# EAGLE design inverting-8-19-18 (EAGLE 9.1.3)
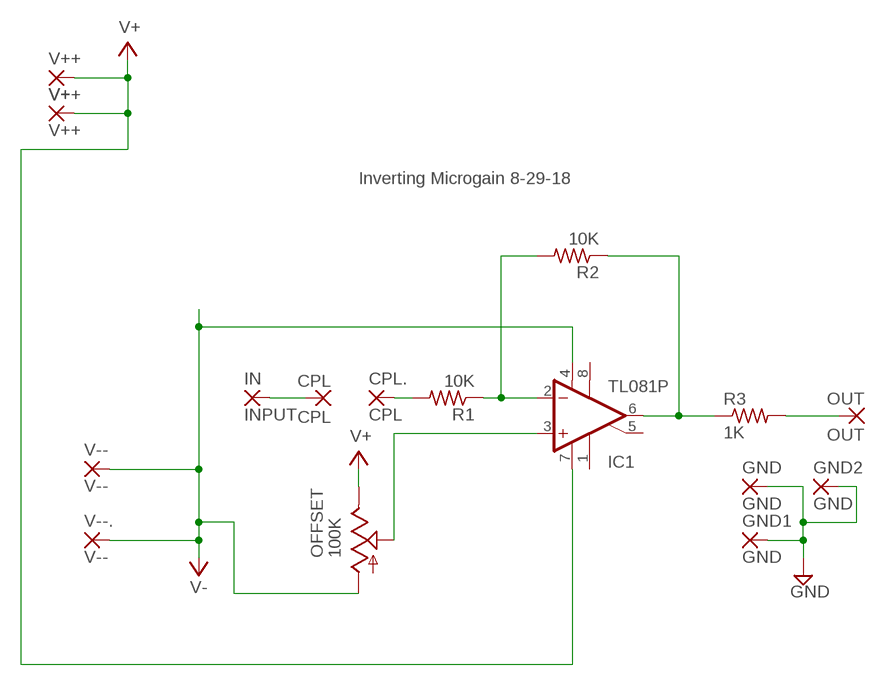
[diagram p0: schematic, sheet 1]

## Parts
CPL  CPL  3,17/1,3  [3,17/1,3]
CPL.  CPL  3,17/1,3  [3,17/1,3]
GND  GND  3,17/1,3  [3,17/1,3]
GND1  GND  3,17/1,3  [3,17/1,3]
GND2  GND  3,17/1,3  [3,17/1,3]
IC1  TL081P  [DIL08]
IN  INPUT  3,17/1,3  [3,17/1,3]
OFFSET  100K  TRIM_US-S63X  [S63X]
OUT  OUT  3,17/1,3  [3,17/1,3]
R1  10K  R-US_0204/7  [0204/7]
R2  10K  R-US_0204/7  [0204/7]
R3  1K  R-US_0204/7  [0204/7]
V+  V++  3,17/1,3  [3,17/1,3]
V++  V++  3,17/1,3  [3,17/1,3]
V--  V--  3,17/1,3  [3,17/1,3]
V--.  V--  3,17/1,3  [3,17/1,3]

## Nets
GND: GND1.1(P) GND2.1(P) GND.1(P)
N$1: IC1.3(+IN) OFFSET.S
N$3: CPL.1(P) IN.1(P)
N$4: CPL..1(P) R1.2
N$5: IC1.2(-IN) R1.1 R2.2
N$18: IC1.6(OUT) R2.1 R3.1
N$19: OUT.1(P) R3.2
V+: IC1.7(V+) OFFSET.E V++.1(P) V+.1(P)
V-: IC1.4(V-) OFFSET.A V--.1(P) V--..1(P)
Unconnected: IC1.1(ON1) IC1.5(ON2) IC1.8(OPT)

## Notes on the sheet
- Inverting Microgain 8-29-18

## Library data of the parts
CPL CPL. GND GND1 GND2 IN OUT V+ V++ V-- V--. = wirepad:3,17/1,3: THROUGH-HOLE PAD
IC1 = linear:TL081: OP AMP
OFFSET = pot:TRIM_US-: POTENTIOMETER
R1-R3 = rcl:R-US_: RESISTOR, American symbol

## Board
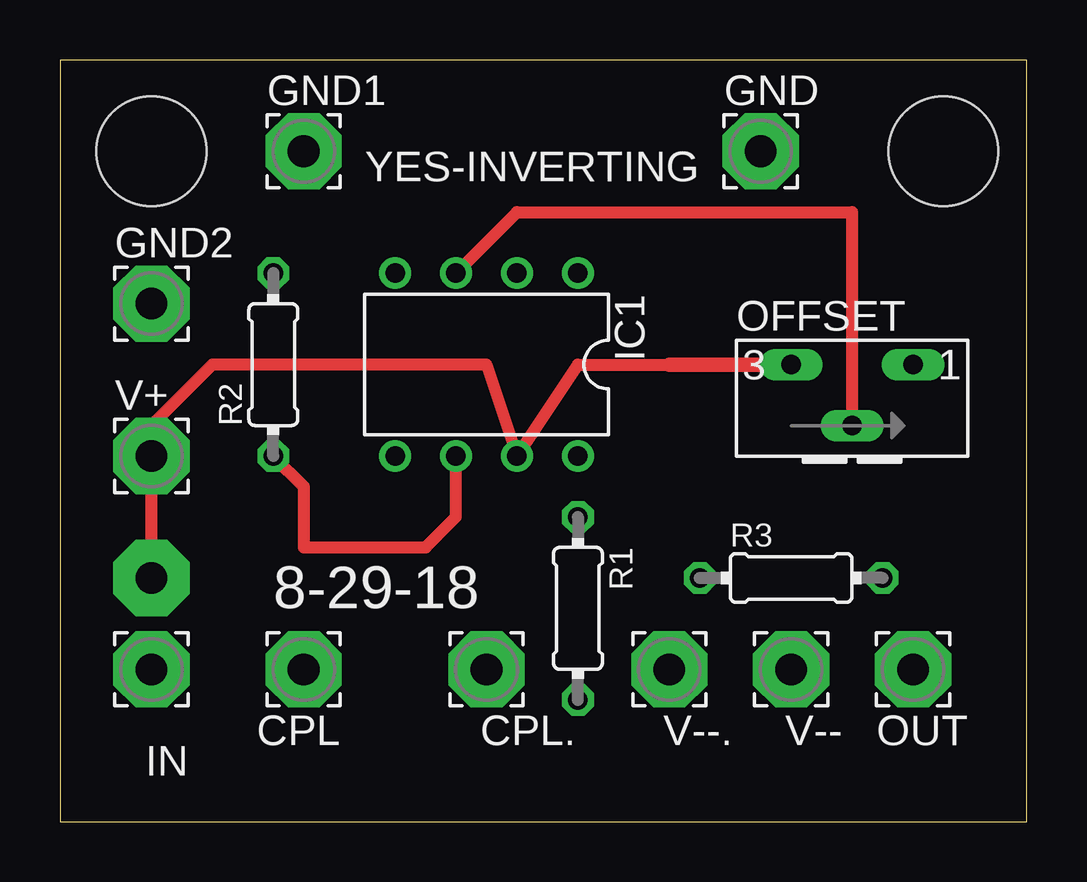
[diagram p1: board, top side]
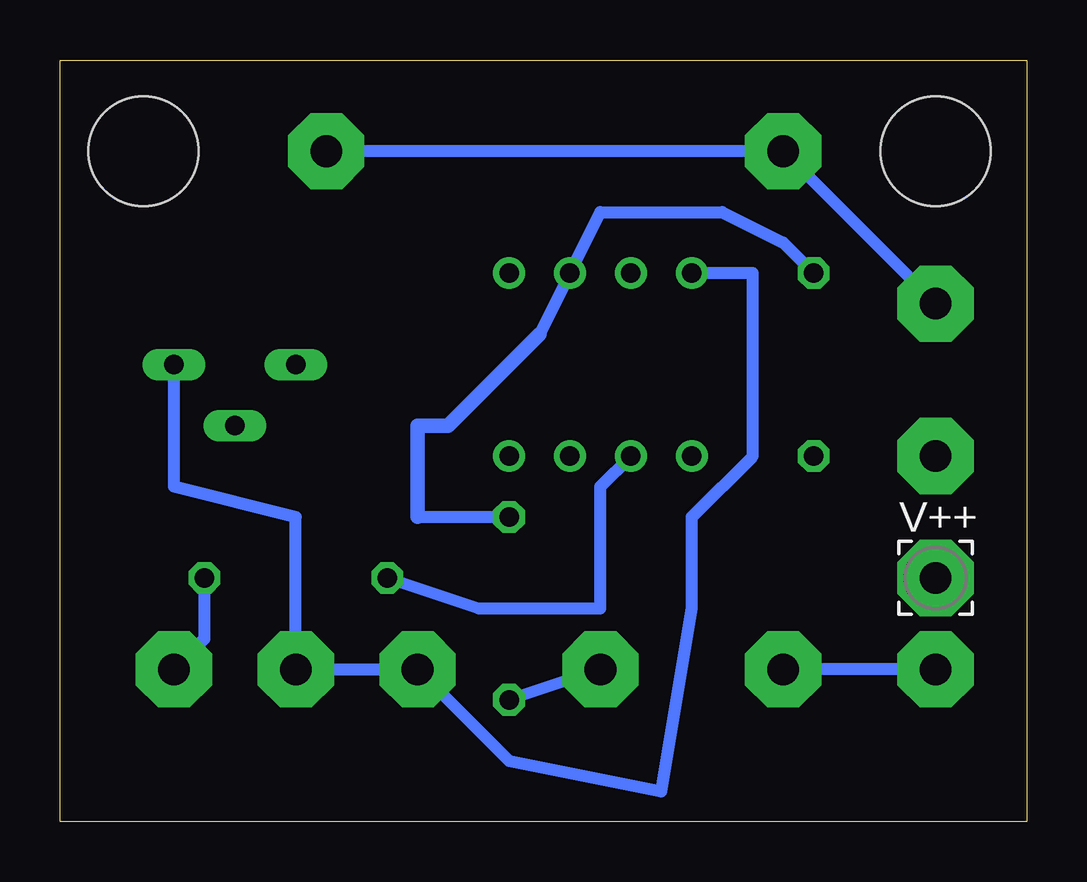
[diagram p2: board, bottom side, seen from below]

Size 40.31 x 31.74 mm. Coordinates in mm from the lower left corner, seen from the top.
Outline: 0,0 40.31,0 40.31,31.74 0,31.74 0,0
Copper layers (1*16): Top 0.035mm / dielectric 1.5mm / Bottom 0.035mm
Design rules "default": minimum track width 6mil, minimum drill 0.35mm, track to track 6mil, track to pad 6mil, pad to pad 6mil, via to via 6mil, smd to smd 6mil, copper to edge 40mil, drill to drill 6mil, minimum pad ring 10mil, minimum via ring 8mil, stop-mask expansion 4mil, vias tented up to drill 0mil, thermal gap 10mil
Holes 4.57 mm at 3.81,27.94 36.83,27.94

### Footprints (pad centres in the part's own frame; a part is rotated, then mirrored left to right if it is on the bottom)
3,17/1,3 = drill 1.321 pad 3.175 octagon: 1 0,0
DIL08 = drill 0.813 pad 1.27: 1 -3.81,-3.81; 2 -1.27,-3.81; 3 1.27,-3.81; 4 3.81,-3.81; 5 3.81,3.81; 6 1.27,3.81; 7 -1.27,3.81; 8 -3.81,3.81
S63X = drill 0.813 long: A 2.54,0; E -2.54,0; S 0,-2.54
0204/7 = drill 0.813 octagon: 1 -3.81,0; 2 3.81,0

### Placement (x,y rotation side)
CPL  10.16,6.35 180 top
CPL.  17.78,6.35 0 top
GND  29.21,27.94 0 top
GND1  10.16,27.94 0 top
GND2  3.81,21.59 0 top
IC1  17.78,19.05 180 top
IN  3.81,6.35 0 top
OFFSET  33.02,19.05 0 top
OUT  35.56,6.35 0 top
R1  21.59,8.89 270 top
R2  8.89,19.05 90 top
R3  30.48,10.16 0 top
V+  3.81,15.24 0 top
V++  3.81,10.16 0 bottom
V--  30.48,6.35 0 top
V--.  25.4,6.35 0 top

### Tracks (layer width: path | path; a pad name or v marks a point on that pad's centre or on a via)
GND
  Bottom 0.508: GND2.1 GND1.1 GND.1
N$1
  Top 0.508: IC1.3 19.05,25.4 33.02,25.4 33.02,20.32 OFFSET.S
N$3
  Bottom 0.508: IN.1 CPL.1
N$4
  Bottom 0.508: CPL..1 R1.2
N$5
  Bottom 0.508: 25.4,12.7 R1.1 | 20.32,20.32 IC1.2 17.78,25.4 12.7,25.4 10.16,24.13 R2.2
  Bottom 0.61: 20.32,20.32 24.13,16.51 25.4,16.51 25.4,12.7
N$18
  Top 0.508: R2.1 10.16,13.97 10.16,11.43 15.24,11.43 16.51,12.7 IC1.6
  Bottom 0.508: R3.1 22.86,8.89 17.78,8.89 17.78,13.97 IC1.6
N$19
  Bottom 0.508: R3.2 34.29,7.62 OUT.1
V+
  Top 0.508: 25.4,19.05 21.59,19.05 IC1.7 17.78,19.05 6.35,19.05 3.81,16.51 V+.1 V++.1
  Top 0.61: 25.4,19.05 OFFSET.E
V-
  Bottom 0.508: IC1.4 11.43,22.86 11.43,15.24 13.97,12.7 13.97,8.89 15.24,1.27 21.59,2.54 V--..1 V--.1 30.48,12.7 35.56,13.97 OFFSET.A

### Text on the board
tNames: YES-INVERTING | 8-29-18
tValues: MICROGAIN!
